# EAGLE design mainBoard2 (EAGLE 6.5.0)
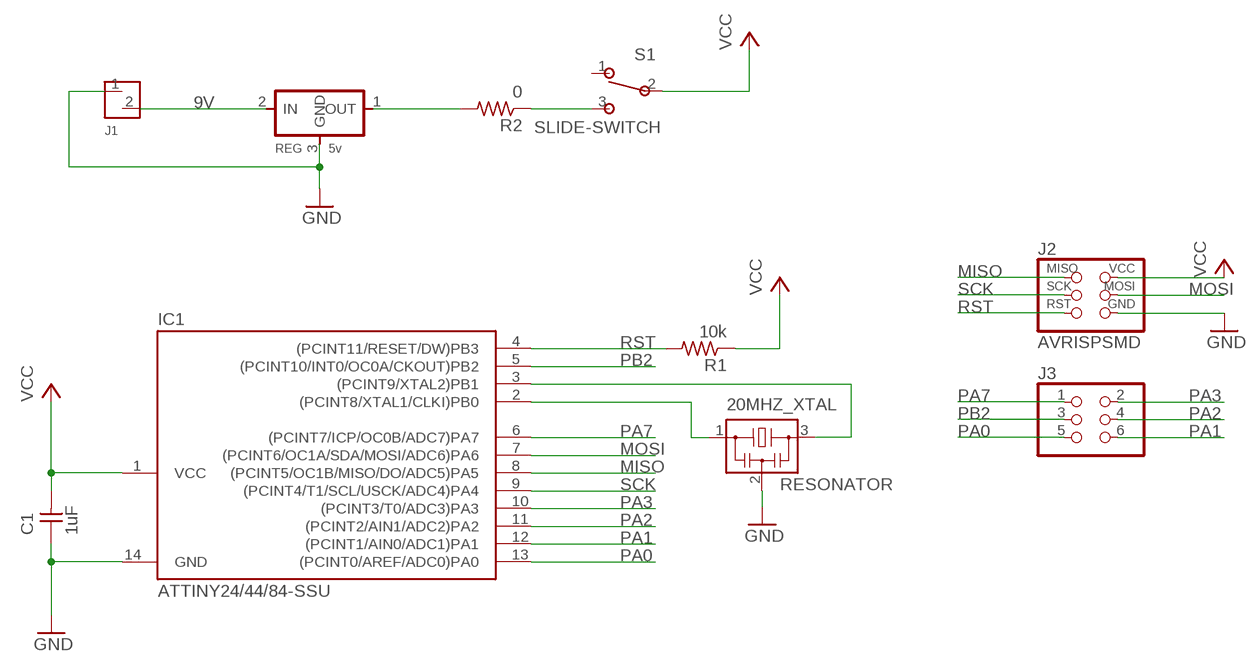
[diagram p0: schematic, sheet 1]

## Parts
20MHZ_XTAL  RESONATOR  [EFOBM]
C1  1uF  UNPOLARIZED_CAPACITOR1206  [1206]
IC1  ATTINY24/44/84-SSU  [SOIC14]
J1  Power  MTA_2MTA_2  [MTA_2]
J2  AVRISPSMD  [2X03SMD]
J3  PINHD-2X3-SMD  [2X03SMD]
R1  10k  RESISTOR1206  [1206]
R2  0  RESISTOR1206  [1206]
REG  5v  REGULATORSOT23  [SOT23]
S1  SLIDE-SWITCH  [AYZ0102AGRLC]

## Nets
9V: J1.2 REG.2(IN)
GND: 20MHZ_XTAL.2 C1.1 IC1.14(GND) J1.1 J2.6(GND) REG.3(GND)
MISO: IC1.8((PCINT5/OC1B/MISO/DO/ADC5)PA5) J2.1(MISO)
MOSI: IC1.7((PCINT6/OC1A/SDA/MOSI/ADC6)PA6) J2.4(MOSI)
N$1: R2.2 REG.1(OUT)
N$2: 20MHZ_XTAL.3 IC1.3((PCINT9/XTAL2)PB1)
N$3: 20MHZ_XTAL.1 IC1.2((PCINT8/XTAL1/CLKI)PB0)
N$4: R2.1 S1.3
PA0: IC1.13((PCINT0/AREF/ADC0)PA0) J3.5
PA1: IC1.12((PCINT1/AIN0/ADC1)PA1) J3.6
PA2: IC1.11((PCINT2/AIN1/ADC2)PA2) J3.4
PA3: IC1.10((PCINT3/T0/ADC3)PA3) J3.2
PA7: IC1.6((PCINT7/ICP/OC0B/ADC7)PA7) J3.1
PB2: IC1.5((PCINT10/INT0/OC0A/CKOUT)PB2) J3.3
RST: IC1.4((PCINT11/RESET/DW)PB3) J2.5(RST) R1.2
SCK: IC1.9((PCINT4/T1/SCL/USCK/ADC4)PA4) J2.3(SCK)
VCC: C1.2 IC1.1(VCC) J2.2(VCC) R1.1 S1.2
Unconnected: S1.1

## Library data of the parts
20MHZ_XTAL = 01_fab:RESONATOR
C1 = 01_FAB_Hello:UNPOLARIZED_CAPACITOR: unpolarized_capacitor
IC1 = 01_attiny24_44_84:ATTINY24/44/84
J1 = 01_ng:MTA_2
J2 = 01_FAB_Hello:AVRISP
J3 = 01_fab:PINHD-2X3-SMD: PIN HEADER
R1 R2 = 01_FAB_Hello:RESISTOR
REG = 01_fab:REGULATOR
S1 = Zaerc:SLIDE-SWITCH

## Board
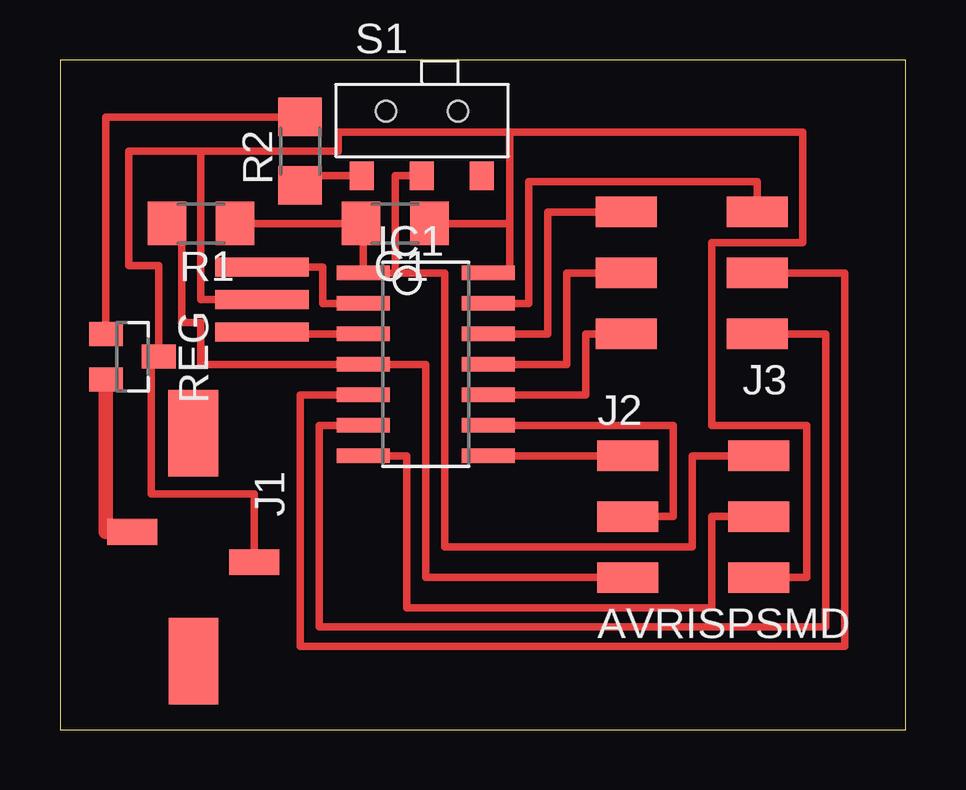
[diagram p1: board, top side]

Size 35.23 x 27.93 mm. Coordinates in mm from the lower left corner, seen from the top.
Outline: 0,0 35.23,0 35.23,27.93 0,27.93 0,0
Copper layers (1*16): Top 0.035mm / dielectric 1.5mm / Bottom 0.035mm
Design rules "default *": minimum track width 10mil, minimum drill 24mil, track to track 0.4mm, track to pad 0.4mm, pad to pad 0.4mm, via to via 0.4mm, smd to smd 0.4mm, copper to edge 40mil, drill to drill 8mil, minimum pad ring 10mil, minimum via ring 8mil, stop-mask expansion 4mil, vias tented up to drill 0mil, thermal gap 10mil

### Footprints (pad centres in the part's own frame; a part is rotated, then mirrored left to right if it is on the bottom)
EFOBM = smd 0.8 x 3.9: 1 -1.35,0; 2 0,0; 3 1.35,0
1206 = smd 1.6 x 1.803: 1 -1.422,0; 2 1.422,0
SOIC14 = smd 0.61 x 2.21: 1 -3.81,-2.603; 2 -2.54,-2.603; 3 -1.27,-2.603; 4 0,-2.603; 5 1.27,-2.603; 6 2.54,-2.603; 7 3.81,-2.603; 8 3.81,2.603; 9 2.54,2.603; 10 1.27,2.603; 11 0,2.603; 12 -1.27,2.603; 13 -2.54,2.603; 14 -3.81,2.603
MTA_2 = smd 1.067 x 2.083: 1 -0.635,-2.54; 2 0.635,2.54 | smd 3.607 x 2.057: P$5 -4.75,0 | smd 3.607 x 2.083: P$6 4.75,0
2X03SMD = smd 2.54 x 1.27: 1 -2.54,2.54; 2 2.92,2.54; 3 -2.54,0; 4 2.92,0; 5 -2.54,-2.54; 6 2.92,-2.54
SOT23 = smd 1 x 1.4: 1 -0.95,-1.1; 2 0.95,-1.1; 3 0,1.1
AYZ0102AGRLC = smd 1 x 1.2: 1 2.5,-2.3; 2 0,-2.3; 3 -2.5,-2.3 | hole 0.85: -1.5,0.4; 1.5,0.4

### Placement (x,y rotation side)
20MHZ_XTAL  8.41,17.94 270 top
C1  13.97,21.11 180 top
IC1  15.24,15.24 270 top
J1  5.56,7.62 90 top
J2  26.19,8.89 0 top
J3  26.51,19.05 180 top
R1  5.87,21.11 180 top
R2  10,24.13 90 top
REG  3.02,15.56 270 top
S1  15.08,25.4 0 top

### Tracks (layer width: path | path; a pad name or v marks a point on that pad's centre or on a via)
9V
  Top 0.61: J1.2 1.92,8.26 REG.2
GND
  Top 0.305: 20MHZ_XTAL.2 5.87,17.94 5.87,24.13 | J2.6 31.11,6.35 31.11,12.7 27.15,12.7 27.15,20.32 30.96,20.32 30.96,24.92 18.73,24.92 | J1.1 8.1,9.84 3.81,9.84 3.81,15.56 REG.3 4.12,19.37 2.86,19.37 2.86,24.13 5.87,24.13 | 5.87,24.13 11.59,24.13 11.59,24.92 18.73,24.92 | IC1.14 18.73,19.05 18.73,21.11 | 18.73,21.11 18.73,24.92 | C1.1 18.73,21.11
MISO
  Top 0.305: J2.1 IC1.8
MOSI
  Top 0.305: J2.4 27.15,8.89 27.15,5.08 14.45,5.08 14.45,11.43 IC1.7
N$1
  Top 0.305: REG.1 1.92,25.55 R2.2
N$2
  Top 0.305: 20MHZ_XTAL.3 8.41,16.51 IC1.3
N$3
  Top 0.305: 20MHZ_XTAL.1 10.95,19.29 10.95,17.78 IC1.2
N$4
  Top 0.305: R2.1 10,23.1 S1.3
PA0
  Top 0.305: IC1.13 19.53,17.78 19.53,22.86 29.05,22.86 J3.5
PA1
  Top 0.305: J3.6 20.32,21.59 20.32,16.51 IC1.12
PA2
  Top 0.305: IC1.11 21.11,15.24 21.11,19.05 J3.4
PA3
  Top 0.305: 17.78,13.97 IC1.10 21.91,13.97 21.91,16.51 J3.2
PA7
  Top 0.305: J3.1 31.91,16.51 31.91,4.29 10.79,4.29 10.79,12.7 IC1.6
PB2
  Top 0.305: J3.3 32.7,19.05 32.7,3.49 10,3.49 10,13.97 IC1.5
RST
  Top 0.305: J2.5 15.24,6.35 15.24,15.24 IC1.4 5.87,15.24 5.87,16.99 5.08,16.99 5.08,21.11 R1.2
SCK
  Top 0.305: J2.3 25.56,8.89 25.56,12.7 IC1.9
VCC
  Top 0.305: J2.2 26.35,11.43 26.35,7.62 16.03,7.62 16.03,19.05 13.97,19.05 | 13.97,19.05 IC1.1 12.64,21.11 C1.2 R1.1 | S1.2 13.97,23.1 13.97,19.05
